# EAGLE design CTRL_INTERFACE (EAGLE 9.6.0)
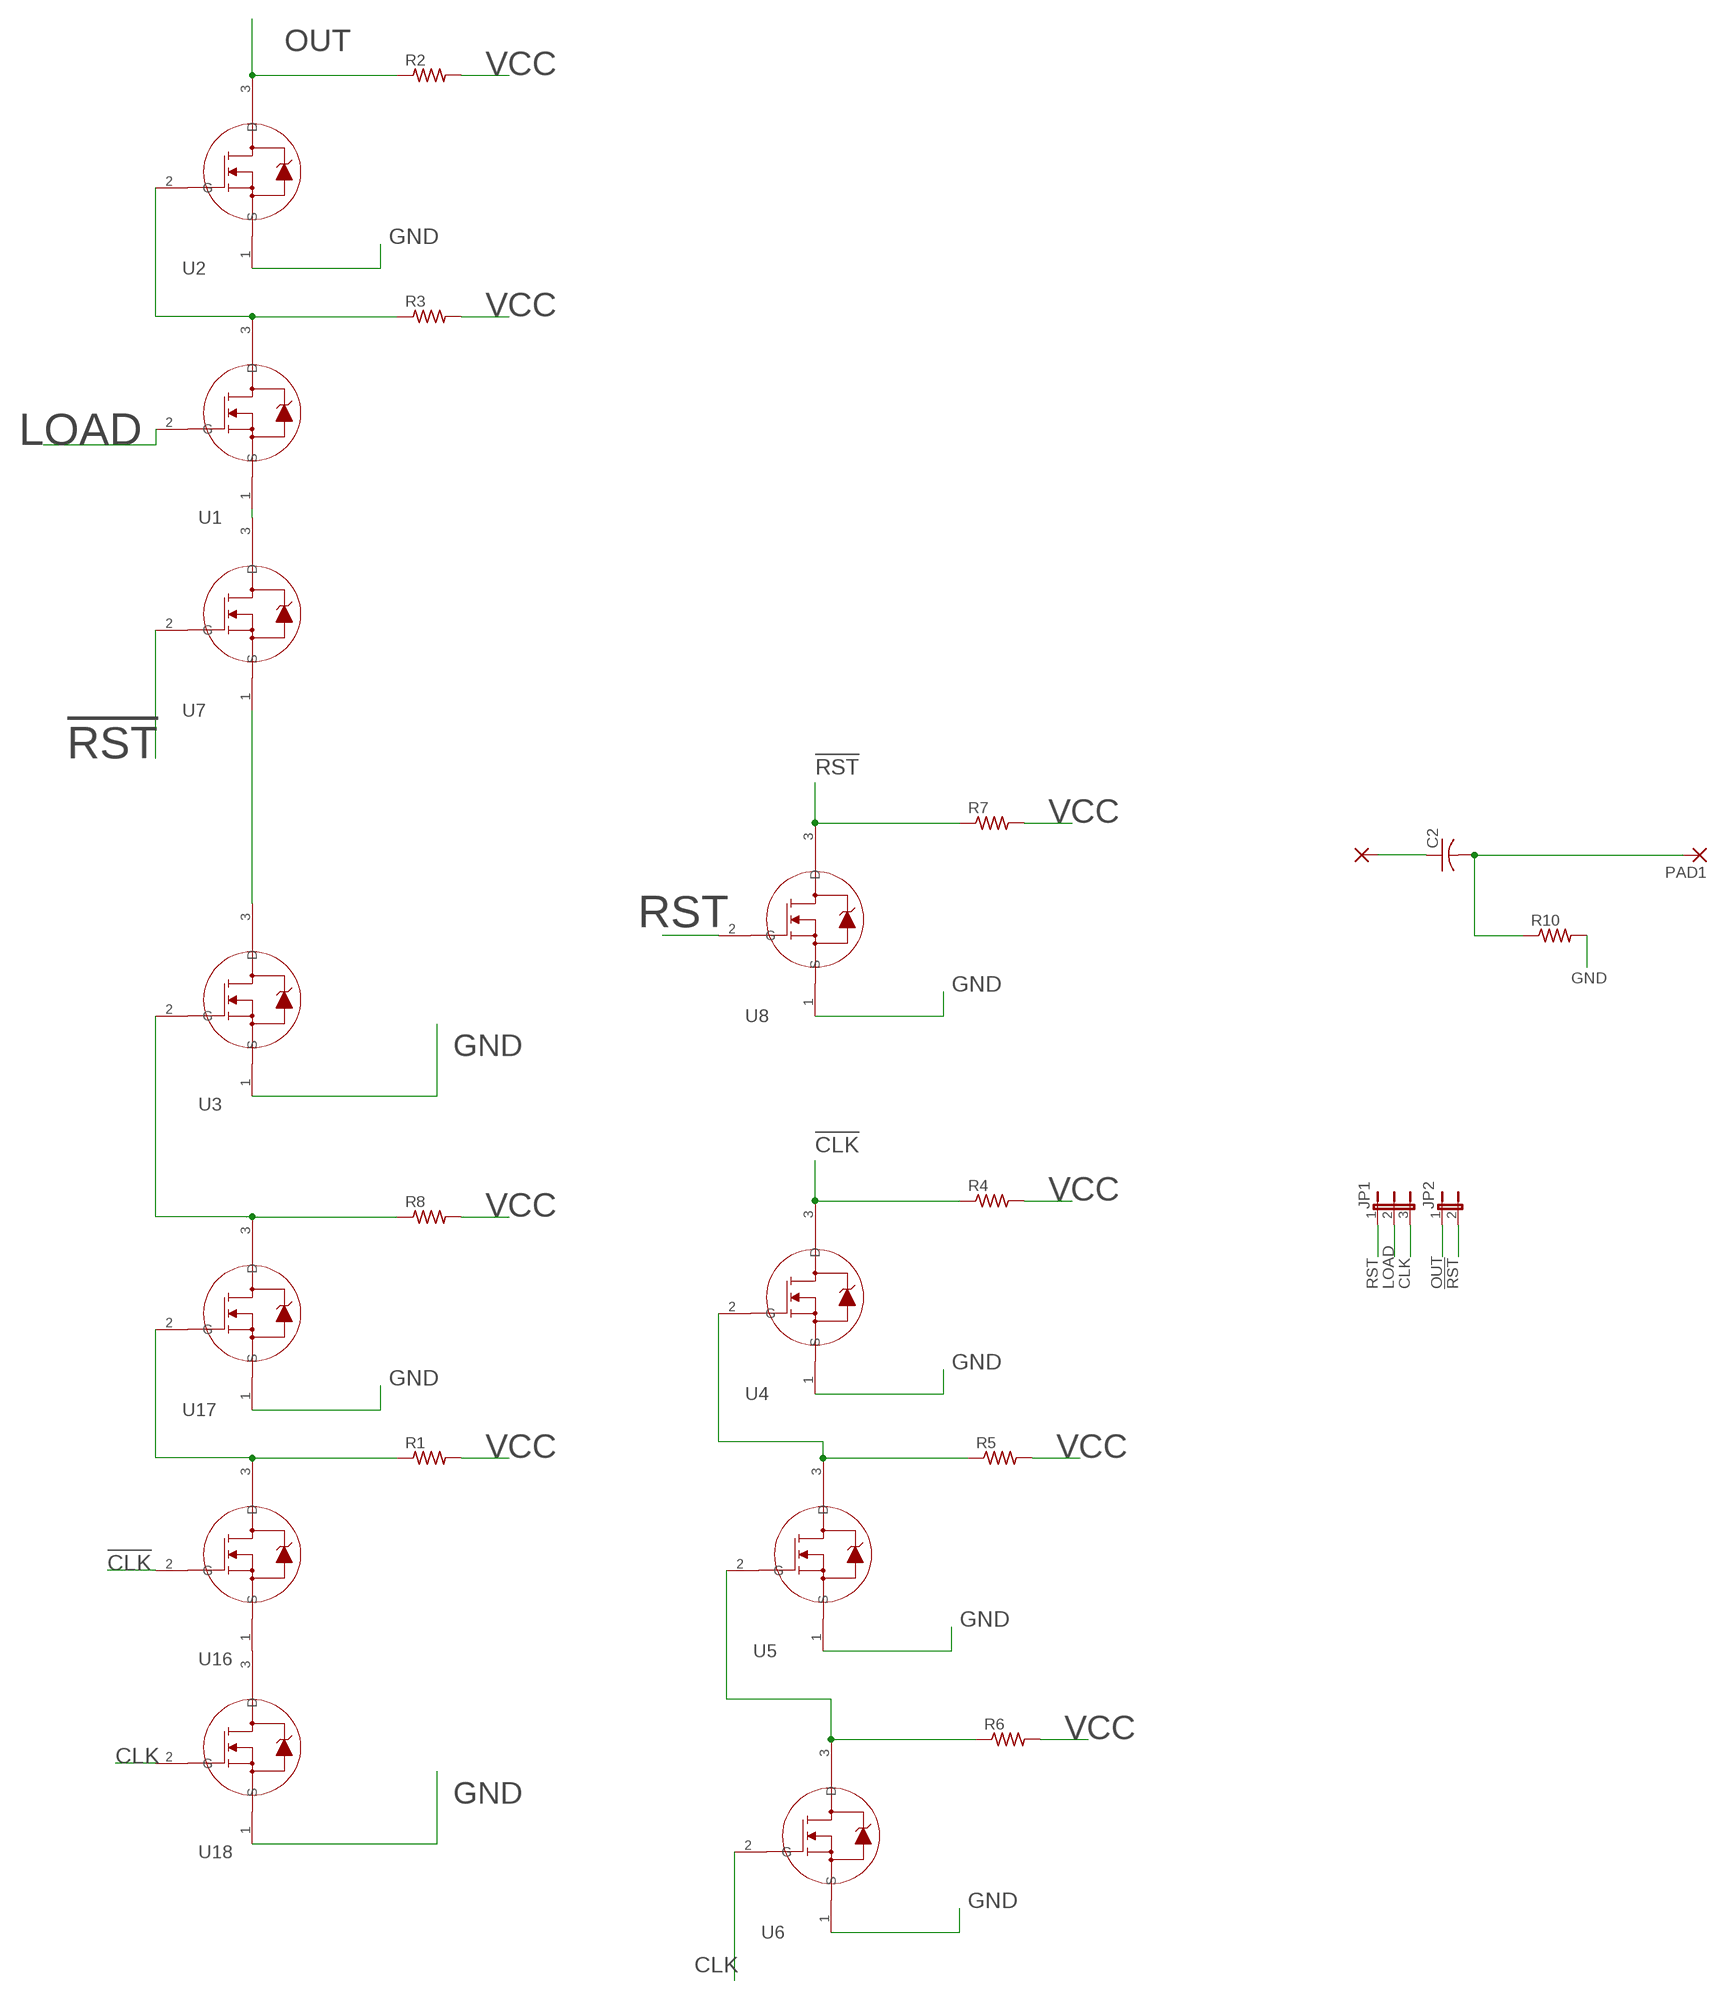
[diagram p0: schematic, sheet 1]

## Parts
C2  C-US050-024X044  [C050-024X044]
JP1  JP2E  [JP2]
JP2  JP1E  [JP1]
PAD1  SMD2  [SMD1,27-2,54]
PAD2  SMD2  [SMD1,27-2,54]
R1  R-US_0204/7  [0204/7]
R2  R-US_0204/7  [0204/7]
R3  R-US_0204/7  [0204/7]
R4  R-US_0204/7  [0204/7]
R5  R-US_0204/7  [0204/7]
R6  R-US_0204/7  [0204/7]
R7  R-US_0204/7  [0204/7]
R8  R-US_0204/7  [0204/7]
R10  R-US_0204/7  [0204/7]
U1  2N7000RLRAG  [TO-92_ONS]
U2  2N7000RLRAG  [TO-92_ONS]
U3  2N7000RLRAG  [TO-92_ONS]
U4  2N7000RLRAG  [TO-92_ONS]
U5  2N7000RLRAG  [TO-92_ONS]
U6  2N7000RLRAG  [TO-92_ONS]
U7  2N7000RLRAG  [TO-92_ONS]
U8  2N7000RLRAG  [TO-92_ONS]
U16  2N7000RLRAG  [TO-92_ONS]
U17  2N7000RLRAG  [TO-92_ONS]
U18  2N7000RLRAG  [TO-92_ONS]

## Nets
!CLK: R4.1 U4.3(D) U16.2(G)
!RST: JP2.2 R7.1 U7.2(G) U8.3(D)
CLK: JP1.3 U6.2(G) U18.2(G)
GND: R10.2 U2.1(S) U3.1(S) U4.1(S) U5.1(S) U6.1(S) U8.1(S) U17.1(S) U18.1(S)
LOAD: JP1.2 U1.2(G)
N$1: R1.1 U16.3(D) U17.2(G)
N$3: U1.1(S) U7.3(D)
N$4: R3.1 U1.3(D) U2.2(G)
N$5: U3.3(D) U7.1(S)
N$6: C2.1 PAD2.1(P)
N$7: R5.1 U4.2(G) U5.3(D)
N$9: R6.1 U5.2(G) U6.3(D)
N$10: C2.2 PAD1.1(P) R10.1
N$17: R8.1 U3.2(G) U17.3(D)
N$18: U16.1(S) U18.3(D)
OUT: JP2.1 R2.1 U2.3(D)
RST: JP1.1 U8.2(G)
VCC: R1.2 R2.2 R3.2 R4.2 R5.2 R6.2 R7.2 R8.2

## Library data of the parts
C2 = rcl:C-US: CAPACITOR, American symbol; SPICEPREFIX: C
JP1 = jumper:JP2E: JUMPER
JP2 = jumper:JP1E: JUMPER
PAD1 PAD2 = wirepad:SMD2: SMD PAD
R1-R8 R10 = rcl:R-US_: RESISTOR, American symbol; SPICEPREFIX: R
U1-U8 U16-U18 = Transistor(MOSFET):2N7000RLRAG; COPYRIGHT: Copyright (C) 2022 Ultra Librarian. All rights reserved.; MANUFACTURER_PART_NUMBER: 2N7000RLRAG; MFR_NAME: onsemi

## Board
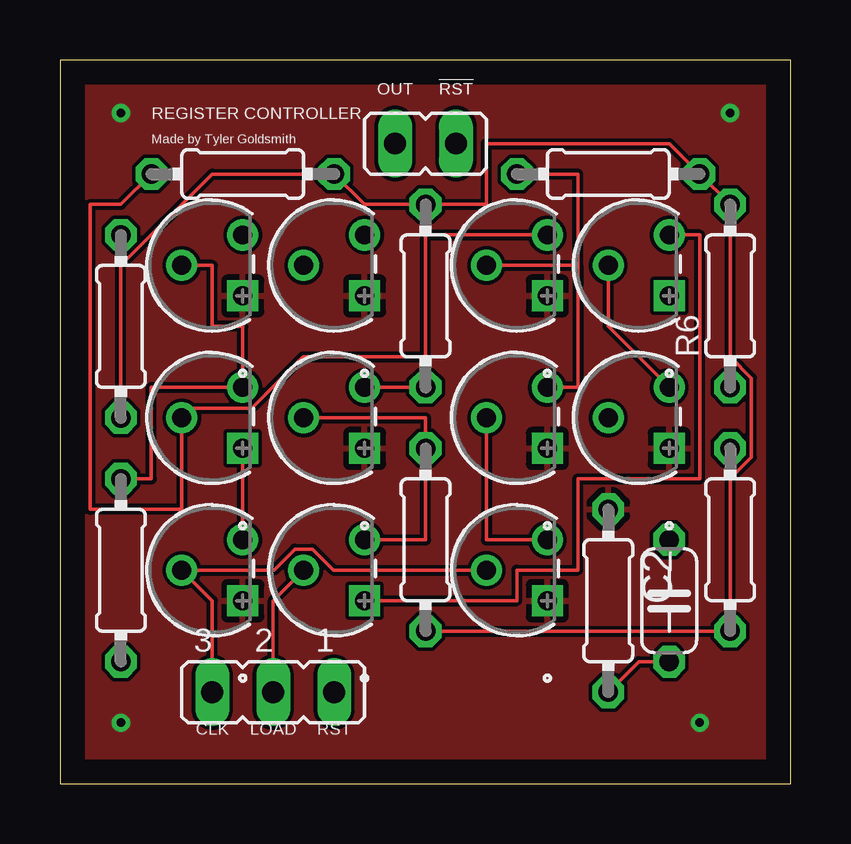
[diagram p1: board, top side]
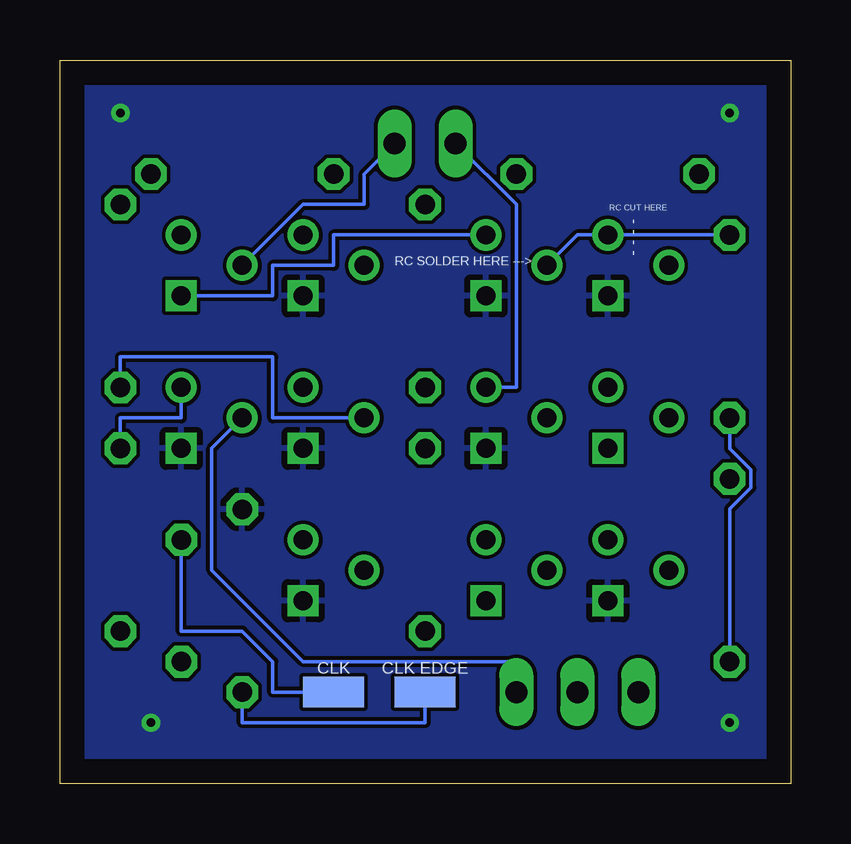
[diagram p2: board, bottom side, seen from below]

Size 30.46 x 30.15 mm. Coordinates in mm from the lower left corner, seen from the top.
Outline: 0,0 30.46,0 30.46,30.15 0,30.15 0,0
Copper layers (1*16): Top 0.035mm / dielectric 1.5mm / Bottom 0.035mm
Design rules "default": minimum track width 6mil, minimum drill 0.35mm, track to track 6mil, track to pad 6mil, pad to pad 6mil, via to via 6mil, smd to smd 6mil, copper to edge 40mil, drill to drill 6mil, minimum pad ring 10mil, minimum via ring 8mil, stop-mask expansion 4mil, vias tented up to drill 0mil, thermal gap 10mil

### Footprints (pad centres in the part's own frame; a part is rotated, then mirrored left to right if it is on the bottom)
C050-024X044 = drill 0.813 octagon: 1 -2.54,0; 2 2.54,0
JP2 = drill 0.914 long: 1 -2.54,0; 2 0,0; 3 2.54,0
JP1 = drill 0.914 long: 1 0,-1.27; 2 0,1.27
SMD1,27-2,54 = smd 1.27 x 2.54: 1 0,0
0204/7 = drill 0.813 octagon: 1 -3.81,0; 2 3.81,0
TO-92_ONS = drill 0.787 pad 1.295 square: 1 0,0 | drill 0.787 pad 1.295: 2 1.27,2.54; 3 2.54,0

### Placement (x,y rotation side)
C2  25.4,7.62 270 top
JP1  8.89,3.81 180 top
JP2  15.24,26.67 270 top
PAD1  15.24,3.81 90 bottom
PAD2  19.05,3.81 90 bottom
R1  2.54,8.89 270 top
R2  15.24,20.32 90 top
R3  15.24,10.16 270 top
R4  7.62,25.4 0 top
R5  22.86,25.4 0 top
R6  27.94,20.32 90 top
R7  27.94,10.16 270 top
R8  2.54,19.05 270 top
R10  22.86,7.62 90 top
U1  12.7,7.62 90 top
U2  12.7,13.97 90 top
U3  12.7,20.32 90 top
U4  20.32,20.32 90 top
U5  20.32,13.97 90 top
U6  20.32,7.62 90 top
U7  25.4,20.32 90 top
U8  25.4,13.97 90 top
U16  7.62,13.97 90 top
U17  7.62,20.32 90 top
U18  7.62,7.62 90 top

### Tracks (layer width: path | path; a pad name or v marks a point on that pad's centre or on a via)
!CLK
  Top 0.152: U4.3 15.24,22.86 15.24,17.78 10.13,17.78 7.98,15.63 5.47,15.63 U16.2 5.08,11.43 1.27,11.43 1.27,24.13 2.54,24.13 R4.1
!RST
  Top 0.152: U8.3 22.86,19.05 U7.2
  Bottom 0.152: U8.3 25.4,15.24 27.94,15.24 R7.1 | U7.2 20.32,24.13 17.78,24.13 17.78,25.4 JP2.2
CLK
  Top 0.152: U6.2 11.4,8.89 10.52,9.77 9.8,9.77 8.92,8.89 U18.2 6.35,7.62 JP1.3
GND  (via drill 0.35)
  other vias: 2.54,27.94 2.54,2.54 26.67,2.54 27.94,27.94
  pour Top: -1.27,31.75 31.75,31.75 31.75,-1.27 0,-1.27 -1.27,0
  pour Bottom: -1.27,31.75 31.75,31.75 31.75,-1.27 0,-1.27 -1.27,0
LOAD
  Top 0.152: JP1.2 8.89,7.62 U1.2
N$1
  Top 0.152: U17.2 6.35,21.59 6.35,19.05 7.62,19.05 U16.3 3.81,16.51 3.81,12.7 R1.1
N$3
  Top 0.152: U1.1 19.05,7.62 19.05,8.89 21.59,8.89 21.59,12.7 26.67,12.7 26.67,22.86 U7.3
N$4
  Top 0.152: U2.2 15.24,15.24 R3.1 15.24,10.16 U1.3
N$5
  Bottom 0.152: U3.3 19.05,22.86 19.05,21.59 21.59,21.59 21.59,20.32 U7.1
N$6
  Bottom 0.152: PAD2.1 21.59,3.81 21.59,5.08 22.86,6.35 25.4,6.35 C2.1
N$7
  Top 0.152: U4.2 21.59,21.59 | 21.59,21.59 21.59,16.51 U5.3 | 21.59,21.59 21.59,25.4 R5.1
N$9
  Top 0.152: U5.2 17.78,10.16 U6.3
  Bottom 0.152: U5.2 21.59,15.24 21.59,17.78 27.94,17.78 R6.1
N$10
  Top 0.152: R10.1 24.13,5.08 C2.2
  Bottom 0.152: PAD1.1 15.24,2.54 22.86,2.54 R10.1
N$17
  Bottom 0.152: R8.1 U17.3 8.89,22.86 U3.2
N$18
  Top 0.152: U18.3 U16.1
OUT
  Top 0.152: R2.1 U2.3
  Bottom 0.152: U2.3 11.43,16.51 11.43,24.13 JP2.1
RST
  Bottom 0.152: JP1.1 11.43,5.08 20.32,5.08 24.13,8.89 24.13,13.97 U8.2
VCC
  Top 0.152: R3.2 R7.2 27.94,12.71 28.83,13.6 28.83,16.89 27.94,17.78 R6.2 R5.2 25.4,26.67 17.78,26.67 17.78,24.13 R2.2 12.7,24.13 R4.2 6.35,25.4 2.54,21.59 R8.2
  Bottom 0.152: R1.2 2.54,11.44 1.65,12.33 1.65,13.07 2.54,13.96 R8.2

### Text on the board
tNames: OUT | !RST | REGISTER CONTROLLER | Made by Tyler Goldsmith | CLK | LOAD | RST
bNames: RC CUT HERE | - - - - | RC SOLDER HERE ---> | CLK EDGE | CLK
